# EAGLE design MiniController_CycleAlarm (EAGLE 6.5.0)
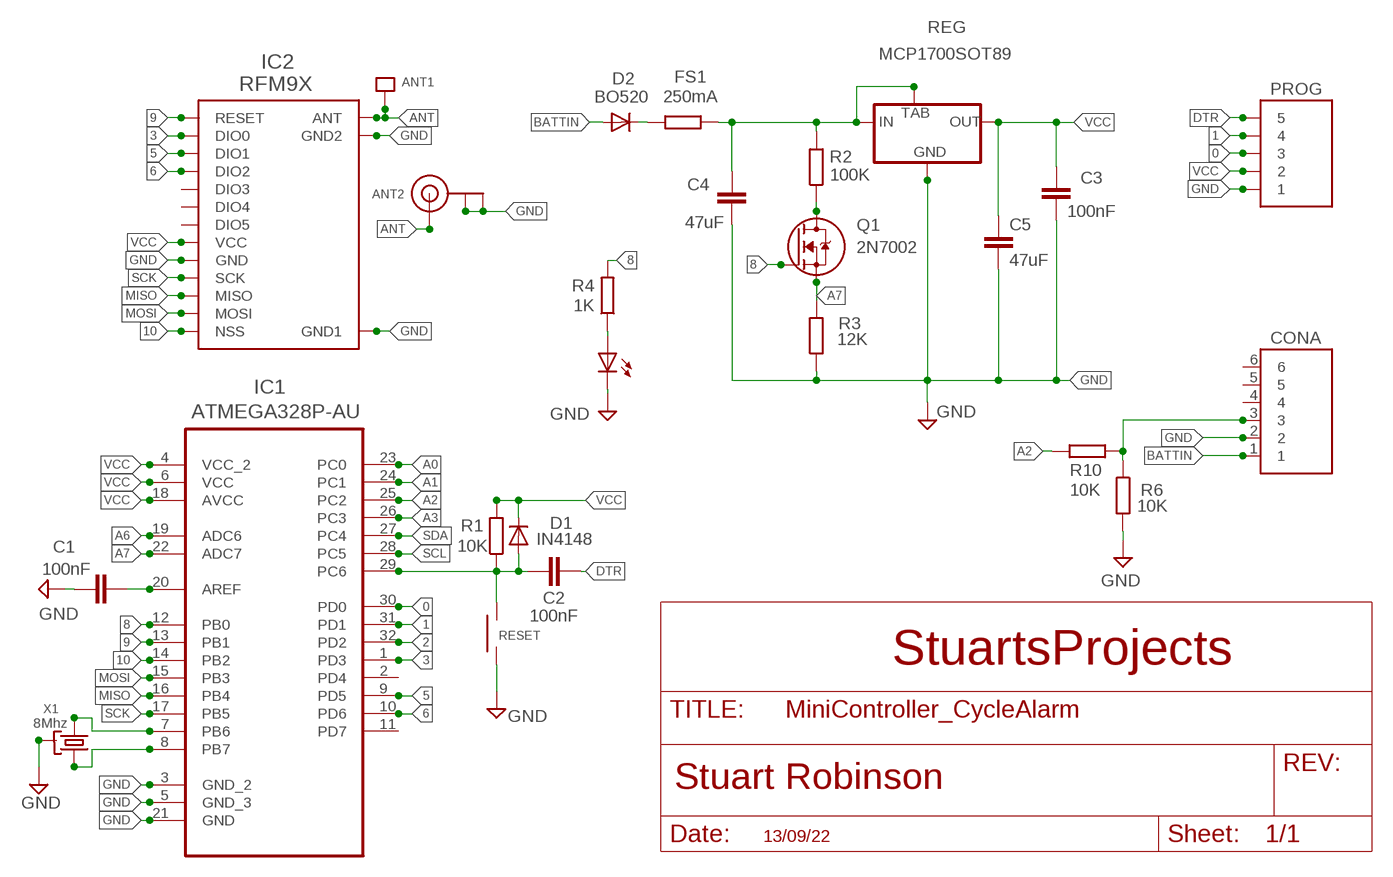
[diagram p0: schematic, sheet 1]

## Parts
ANT1  SINGLEPAD  [SINGLEPAD]
ANT2  ANTENNA_U.FL  [U.FL]
C1  100nF  C805_REDUCED  [C0805_REDUCED]
C2  100nF  C805_REDUCED  [C0805_REDUCED]
C3  100nF  C805_REDUCED  [C0805_REDUCED]
C4  47uF  C-EUC1206  [C1206]
C5  47uF  C-EUC1206  [C1206]
CONA  6X1BATPADS  [6X1_BATPADS]
D1  IN4148  DIODE-SOD123  [SOD123]
D2  BO520  DIODE-SOD123  [SOD123]
FS1  250mA  R-EU_R1206  [R1206]
IC1  ATMEGA328P-AU  [QFP80P900X900X120-32N]
IC2  RFM9X  RFM98  [RFM98]
L1  RED  LEDCHIPLED_0805  [CHIPLED_0805]
PROG  5X1  [5X1]
Q1  2N7002  [SOT23]
R1  10K  R0805_REDUCED  [R0805_REDUCED]
R2  100K  R0805_REDUCED  [R0805_REDUCED]
R3  12K  R0805_REDUCED  [R0805_REDUCED]
R4  1K  R0805_REDUCED  [R0805_REDUCED]
R6  10K  R0805_REDUCED  [R0805_REDUCED]
R10  10K  R0805_REDUCED  [R0805_REDUCED]
REG  MCP1700SOT89  [MCP1700SOT89]
RESET  SMTSWITCH_4_X_3  [SMTSWITCH_4_X_3]
X1  8Mhz  SMTRESONATOR3  [SMTRESONATOR3]

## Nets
0: IC1.30(PD0) PROG.3
1: IC1.31(PD1) PROG.4
2: IC1.32(PD2)
3: IC1.1(PD3) IC2.14(DIO0)
5: IC1.9(PD5) IC2.15(DIO1)
6: IC1.10(PD6) IC2.16(DIO2)
8: IC1.12(PB0) Q1.1(G) R4.2
9: IC1.13(PB1) IC2.6(RESET)
10: IC1.14(PB2) IC2.5(NSS)
A0: IC1.23(PC0)
A1: IC1.24(PC1)
A2: IC1.25(PC2) R10.2
A3: IC1.26(PC3)
A6: IC1.19(ADC6)
A7: IC1.22(ADC7) Q1.2(S) R3.2
ANT: ANT1.P$1 ANT2.3(SIGNAL) IC2.9(ANT)
BATTIN [POWER]: CONA.1 D2.A
DTR: C2.2 PROG.5
GND [POWER]: ANT2.1(GND) ANT2.2(GND) C1.2 C3.2 C4.2 C5.2 CONA.2 IC1.3(GND_2) IC1.5(GND_3) IC1.21(GND) IC2.1(GND) IC2.8(GND1) IC2.10(GND2) L1.C PROG.1 R3.1 R6.2 REG.1(GND) RESET.1 X1.G(GND)
MISO: IC1.16(PB4) IC2.2(MISO)
MOSI: IC1.15(PB3) IC2.3(MOSI)
N$2: IC1.8(PB7) X1.X1
N$3: C1.1 IC1.20(AREF)
N$5 [POWER]: D2.C FS1.2
N$6: L1.A R4.1
N$9: Q1.3(D) R2.1
N$11 [POWER]: C4.1 FS1.1 R2.2 REG.2(IN) REG.4(TAB)
N$13: CONA.3 R6.1 R10.1
N$16: IC1.7(PB6) X1.X2
RESET: C2.1 D1.A IC1.29(PC6) R1.1 RESET.2
SCK: IC1.17(PB5) IC2.4(SCK)
SCL: IC1.28(PC5)
SDA: IC1.27(PC4)
VCC [VDD]: C3.1 C5.1 D1.C IC1.4(VCC_2) IC1.6(VCC) IC1.18(AVCC) IC2.13(VCC) PROG.2 R1.2 REG.3(OUT)
Unconnected: CONA.4 CONA.5 CONA.6 IC1.2(PD4) IC1.11(PD7) IC2.7(DIO5) IC2.11(DIO3) IC2.12(DIO4)

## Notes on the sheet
- StuartsProjects
- 13/09/22

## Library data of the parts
ANT1 = LMA2:SINGLEPAD
ANT2 = adafruit:ANTENNA_U.FL: U.FL Antenna Connector
C1-C3 = resistor:C805_REDUCED
C4 C5 = resistor:C-EU: CAPACITOR, European symbol
CONA = My_Pin_Headers:6X1
D1 D2 = diode:DIODE-: DIODE
FS1 = resistor:R-EU_: RESISTOR, European symbol
IC1 = atmel:ATMEGA328P-AU: 8-bit Microcontroller with In-System Programmable Flash; MPN: ATMEGA328P-AU; OC_FARNELL: 1715486; OC_NEWARK: 14R4631; PACKAGE: TQFP-32; SUPPLIER: Atmel
IC2 = LMA2:RFM98
L1 = led:LED: LED
PROG = My_Pin_Headers:5X1
Q1 = LMA2:2N7002
R1-R4 R6 R10 = resistor:R0805_REDUCED
REG = LMA2:MCP1700SOT89
RESET = LMA2:SMTSWITCH_4_X_3
X1 = LMA2:SMTRESONATOR3

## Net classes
0 default: width 0.152 mm
1 POWER: width 0.508 mm
2 VDD: width 0.508 mm
3 gpspower: width 0.508 mm

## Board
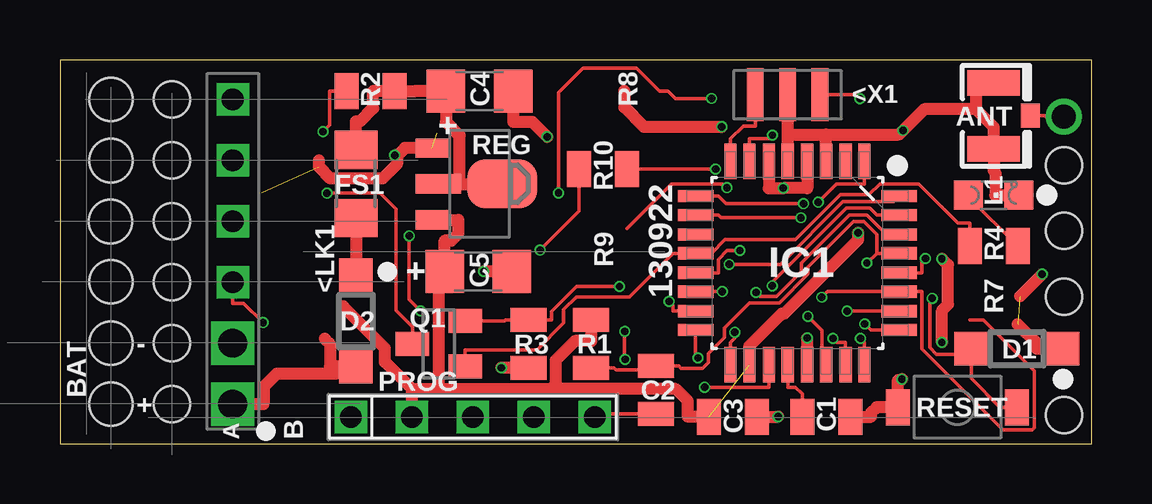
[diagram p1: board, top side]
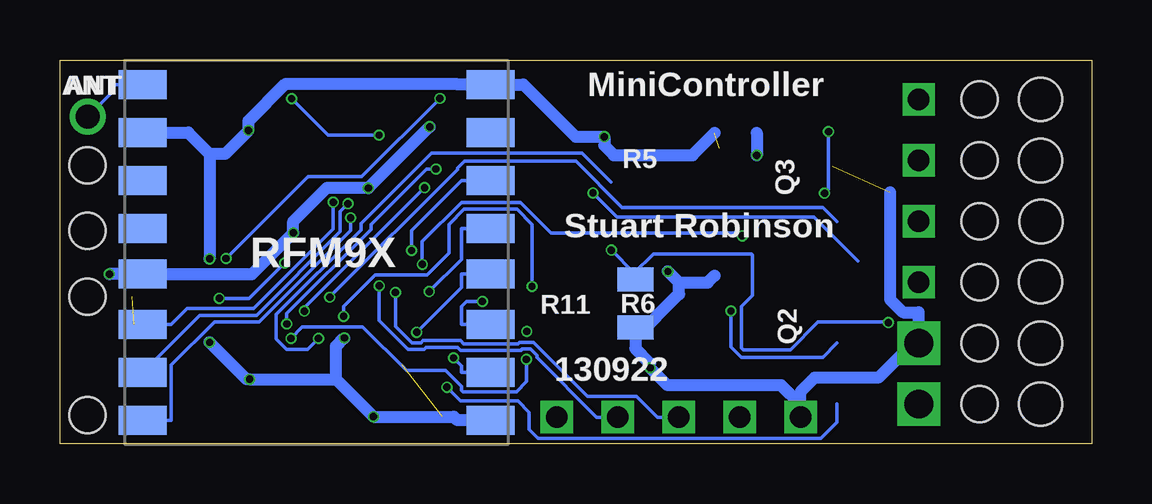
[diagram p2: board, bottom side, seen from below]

Size 43 x 16 mm. Coordinates in mm from the lower left corner, seen from the top.
Outline: 0,0 43,0 43,16 0,16 0,0
Copper layers (1*16): Top 0.035559375mm / dielectric 1.6mm / Bottom 0.035559375mm
Design rules "jlcpcb2layer *": minimum track width 5mil, minimum drill 12mil, track to track 5mil, track to pad 5mil, pad to pad 5mil, via to via 5mil, smd to smd 5mil, copper to edge 8mil, drill to drill 6mil, minimum pad ring 5mil, minimum via ring 3mil, stop-mask expansion 2.5mil, vias tented up to drill 1000mil, thermal gap 10mil
Holes 1.5 mm at 41.85,11.61 41.85,6.13 41.85,1.18 41.85,8.87 4.66,14.35 4.66,11.81 4.66,9.27 4.66,6.73 4.66,4.19 4.66,1.65
Holes 1.8 mm at 2.12,14.35 2.12,11.8 2.11,9.26 2.12,6.75 2.12,4.19 2.12,1.65
tRestrict: area 0,0 to 6.4,16
bRestrict: area 41.4,17.3 to 41.4,17.3; area 0,-0.1 to 6.4,16

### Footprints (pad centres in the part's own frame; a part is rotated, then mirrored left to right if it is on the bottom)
SINGLEPAD = drill 1: P$1 0,0
U.FL = smd 2.2 x 1.05: 1 0,1.375; 2 0,-1.375 | smd 0.8 x 1: 3 1.525,0
C0805_REDUCED = smd 1 x 1.5: 1 -1,0; 2 1,0
C1206 = smd 1.6 x 1.8: 1 -1.4,0; 2 1.4,0
6X1_BATPADS = drill 1.2 square: 1 -6.35,0; 2 -3.81,0 | drill 0.9 square: 3 -1.27,0; 4 1.27,0; 5 3.81,0; 6 6.35,0
SOD123 = smd 1.4 x 1.4: A 1.9,0; C -1.9,0
R1206 = smd 1.6 x 1.803: 1 -1.422,0; 2 1.422,0
QFP80P900X900X120-32N = smd 1.473 x 0.508: 1 -4.242,2.794; 2 -4.242,2.007; 3 -4.242,1.194; 4 -4.242,0.406; 5 -4.242,-0.406; 6 -4.242,-1.194; 7 -4.242,-2.007; 8 -4.242,-2.794; 17 4.242,-2.794; 18 4.242,-2.007; 19 4.242,-1.194; 20 4.242,-0.406; 21 4.242,0.406; 22 4.242,1.194; 23 4.242,2.007; 24 4.242,2.794 | smd 0.508 x 1.473: 9 -2.794,-4.242; 10 -2.007,-4.242; 11 -1.194,-4.242; 12 -0.406,-4.242; 13 0.406,-4.242; 14 1.194,-4.242; 15 2.007,-4.242; 16 2.794,-4.242; 25 2.794,4.242; 26 2.007,4.242; 27 1.194,4.242; 28 0.406,4.242; 29 -0.406,4.242; 30 -1.194,4.242; 31 -2.007,4.242; 32 -2.794,4.242
RFM98 = smd 2 x 1.2: 1 -7.25,7; 2 -7.25,5; 3 -7.25,3; 4 -7.25,0.9; 5 -7.25,-1; 6 -7.25,-3; 7 -7.25,-5; 8 -7.25,-7; 9 7.25,-7; 10 7.25,-5; 11 7.25,-3; 12 7.25,-1; 13 7.25,0.9; 14 7.25,3; 15 7.25,5; 16 7.25,7
CHIPLED_0805 = smd 1.2 x 1.2: A 0,-1.05; C 0,1.05
5X1 = drill 0.9 square: 1 -5.08,0; 2 -2.54,0; 3 0,0; 4 2.54,0; 5 5.08,0
SOT23 = smd 1 x 1.4: 1 -0.95,-1.1; 2 0.95,-1.1; 3 0,1.1
R0805_REDUCED = smd 1 x 1.5: 1 -1,0; 2 1,0
MCP1700SOT89 = smd 0.8 x 1.4: 1 -1.499,-1.981; 3 1.499,-1.981 | smd 0.8 x 1.9: 2 0,-1.727 | smd 2.032 x 2.921: 4 0,0.94
SMTSWITCH_4_X_3 = smd 1 x 1.5: 1 -2.48,0; 2 2.48,0
SMTRESONATOR3 = smd 0.7 x 2.2: G 0,0; X1 -1.35,0; X2 1.35,0

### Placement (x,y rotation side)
ANT1  41.85,13.63 0 top
ANT2  38.92,13.67 0 top
C1  31.94,1.12 0 top
C2  24.84,2.24 270 top
C3  28.05,1.12 0 top
C4  17.49,14.7 0 top
C5  17.44,7.18 0 top
CONA  7.2,8 90 top
D1  39.89,3.96 180 top
D2  12.34,5.11 270 top
FS1  12.34,10.83 270 top
IC1  30.74,7.53 270 top
IC2  32.31,7.97 180 bottom
L1  38.92,10.36 270 top
PROG  17.21,1.1 0 top
Q1  15.79,4.16 90 top
R1  22.14,4.16 90 top
R2  12.94,14.7 0 top
R3  19.53,4.16 90 top
R4  38.92,8.24 180 top
R6  19.02,5.85 270 bottom
R10  22.64,11.45 0 top
REG  17.5,10.83 270 top
RESET  37.41,1.52 0 top
X1  30.33,14.55 0 top

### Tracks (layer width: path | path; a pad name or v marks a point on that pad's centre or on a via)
0  (via drill 0.3 pad 0.46)
  Top 0.152: IC1.30 34.46,8.72 33.64,9.54 32.92,9.54 30.91,7.53 30.91,7.18 29.87,6.14 29.18,6.14 v29.02,6.3
  Bottom 0.152: 21.02,1.98 18.97,1.98 18.09,1.1 PROG.3 | 21.02,1.98 | 21.02,1.98 23.26,4.22 23.85,4.22 23.91,4.17 26.18,4.17 26.31,4.3 27.86,4.3 27.95,4.21 28.33,4.21 29.02,4.89 v29.02,6.3
1  (via drill 0.3 pad 0.46)
  Top 0.152: v29.69,6.58 29.69,6.73 32.78,9.82 33.76,9.82 34.04,9.54 IC1.31
  Bottom 0.152: v29.69,6.58 29.69,5.14 28.48,3.93 27.83,3.93 27.74,4.02 26.43,4.02 26.29,3.88 23.79,3.88 23.73,3.94 23.38,3.94 23.12,3.69 23.12,3.6 20.63,1.1 PROG.4
2  (via drill 0.3 pad 0.46)
  Top 0.152: v27.9,7.48 30.02,7.48 32.64,10.1 34.75,10.1 IC1.32 | v15.03,5.53 14.56,6 v14.56,8.66
  Bottom 0.152: v14.56,8.66 14.67,8.78 22.54,8.78 23.81,10.05 26.26,10.05 27.9,8.42 v27.9,7.48 | 10.62,4.19 11.21,3.6 14.6,3.6 15.03,4.04 v15.03,5.53
3  (via drill 0.3 pad 0.46)
  Top 0.152: v31.61,10.07 32.37,10.83 33.53,10.83 IC1.1
  Bottom 0.152: v31.61,10.07 31.61,8.94 34.92,5.63 37.7,5.63 38.36,4.97 IC2.14
5  (via drill 0.3 pad 0.46)
  Top 0.152: IC1.9 27.44,10.32 27.76,10 v31,10
  Bottom 0.152: IC2.15 37.18,5.35 34.81,5.35 31.31,8.84 31.31,9.68 v31,10
6  (via drill 0.3 pad 0.46)
  Top 0.152: v30.88,9.42 27.56,9.42 27.44,9.54 IC1.10
  Bottom 0.152: v30.88,9.42 30.88,8.88 34.69,5.07 36.56,5.07 38.36,3.27 38.36,0.97 IC2.16
8
  Top 0.152: Q1.1 16.89,3.91 19.89,3.91 21,5.02 21,5.59 21.53,6.12 23.74,6.12 25.56,7.94 IC1.12 27.16,7.94 27.72,8.5 30.65,8.5 32.53,10.38 33.73,10.38 34.18,10.83 35.8,10.83 37.44,9.19 37.92,9.19 R4.2
9  (via drill 0.3 pad 0.46)
  Top 0.152: v28.34,8.05 27.8,8.05 27.44,7.68 27.44,7.12 IC1.13
  Bottom 0.152: v28.34,8.05 28.34,8.89 26.26,10.97 IC2.6
10  (via drill 0.3 pad 0.46)
  Top 0.152: v27.61,6.34 27.44,6.34 IC1.14
  Bottom 0.152: v27.61,6.34 26.26,7.68 26.26,8.97 IC2.5
A0  (via drill 0.3 pad 0.46)
  Top 0.152: v32.22,4.38 32.38,4.23 32.75,4.23 IC1.23
  Bottom 0.152: v32.22,4.38 32.68,3.93 33.55,3.93 33.98,4.37 33.98,5.38 30.45,8.91 30.45,9.17 27.51,12.11 21.24,12.11 20.04,10.91
A1  (via drill 0.3 pad 0.46)
  Top 0.152: v23.54,4.68 23.54,3.52 v23.56,3.51 | v33.37,4.39 33.53,4.23 IC1.24
  Bottom 0.152: 23.42,4.8 v23.54,4.68 | v23.56,3.51 23.56,2.59 23.98,2.17 26.2,2.17 26.26,2.23 26.26,2.38 26.93,3.04 28.56,3.04 30.38,4.86 32.9,4.86 v33.37,4.39
A2  (via drill 0.3 pad 0.46)
  Top 0.152: R10.2 v27.33,11.45 | v33.55,4.99 33.8,4.74 IC1.25
  Bottom 0.152: v33.55,4.99 33.55,5.42 30.03,8.94 30.03,9.13 27.72,11.45 v27.33,11.45
A3  (via drill 0.3 pad 0.46)
  Top 0.152: 23.64,8.97 25.5,10.83 27.64,10.83 v27.8,10.67 | v32.81,5.52 IC1.26
  Bottom 0.152: v32.81,5.52 32.81,5.66 v27.8,10.67
A6  (via drill 0.3 pad 0.46)
  Top 0.152: v26.87,2.35 29.55,2.35 IC1.19
  Bottom 0.152: 10.62,1.65 10.62,0.88 11.28,0.22 23.08,0.22 23.45,0.6 23.45,1.31 23.91,1.77 26.29,1.77 v26.87,2.35
A7  (via drill 0.3 pad 0.46)
  Top 0.152: v31.18,5.31 31.77,4.72 31.77,3.45 IC1.22 | v23.32,6.56 21.53,6.56 20.48,5.51 20.48,5.16 R3.2 19.05,5.16 18.58,5.16 18.53,5.11 Q1.2
  Bottom 0.152: v23.32,6.56 23.32,9.14 23.96,9.77 26.15,9.77 26.78,9.14 26.78,7.95 27.71,7.03 29.87,7.03 31.18,5.72 v31.18,5.31
ANT
  Top 0.152: ANT1.P$1 41.09,13.63 41.05,13.67 ANT2.3
  Bottom 0.152: IC2.9 40.76,14.97 40.76,14.72 ANT1.P$1
BATTIN
  Top 0.508: CONA.1 8.48,1.65 8.48,2.36 9.03,2.91 11.5,2.91 11.8,3.21 | 11.8,3.21 11.26,3.21 11.26,4.15 11.04,4.37 | D2.A 11.8,3.21
DTR
  Top 0.152: PROG.5 22.43,1.24 23.89,1.24 C2.2
GND  (via drill 0.3 pad 0.46)  (2 unrouted)
  Top 0.508: IC1.21 v31.15,4.41 | C3.2 v29.93,1.12 | C5.2 v17.66,7.18 | v20.31,12.79 19.68,13.42 18.89,13.42 C4.2 | 14.04,12 14.04,11.65 13.46,11.06 11.28,11.06 10.8,11.54 10.8,11.81 | 14.04,12 14.38,12.33 14.44,12.33 REG.1 | 14.04,12 14.01,12.03 v13.95,12.03 | v36.76,4.22 36.76,5.55 37.02,5.81 37.02,7.45 v36.76,7.71 | 30.33,12.89 30.33,13.06 30.33,13.07 X1.G | IC1.5 30.33,12.89 | 30.33,12.89 31.93,12.89 | 31.93,12.89 34.97,12.89 v35.14,13.06 36.02,13.94 38.18,13.94 | C1.2 33.82,1.12 33.82,1.29 34.05,1.52 RESET.1 34.93,2.65 35.06,2.65 v35.09,2.68 | IC1.3 31.93,12.89 | L1.C 38.99,10.36 38.99,11.32 38.92,11.39 ANT2.2 38.92,13.2 38.18,13.94 | ANT2.1 38.18,15.04 38.18,13.94 | R3.1 v18.4,3.16
  Bottom 0.508: 15.71,12.95 16.63,12.03 19.91,12.03 20.31,12.43 v20.31,12.79 21.5,12.79 23.68,14.97 IC2.8 26.44,14.97 26.48,15.01 33.59,15.01 35.14,13.45 v35.14,13.06 36.12,12.08 36.76,12.08 | 31.5,2.68 31.5,4.06 v31.15,4.41 | 31.5,2.68 v29.93,1.12 26.59,1.12 26.44,0.97 IC2.1 | 31.5,2.68 v35.09,2.68 35.23,2.68 v36.76,4.22 | 17.19,6.71 v17.66,7.18 | 19.02,4.41 17.19,6.24 17.19,6.71 | 17.19,6.71 16.01,6.71 15.71,7.01 | 19.02,4.41 19.02,3.97 18.4,3.35 v18.4,3.16 17.68,2.44 12.94,2.44 12.13,1.63 | R6.2 19.02,4.41 | 12.13,1.63 12.13,2.16 11.54,2.74 8.89,2.74 7.2,4.43 | PROG.1 12.13,1.63 | 13.95,12.95 v13.95,12.03 | CONA.2 7.2,4.43 | 7.2,4.43 7.2,4.47 7.2,5.47 7.86,5.47 8.4,6.02 8.4,10.47 | IC2.10 37.65,12.97 36.76,12.08 | 36.76,12.08 v36.76,7.71
MISO  (via drill 0.3 pad 0.46)
  Top 0.152: IC1.16 26.5,3.67 v26.59,3.57
  Bottom 0.152: v26.59,3.57 26.26,3.24 26.26,2.97 IC2.2
MOSI  (via drill 0.3 pad 0.46)
  Top 0.152: IC1.15 25.56,5.52 25.56,5.76 v25.39,5.93
  Bottom 0.152: IC2.3 26.26,4.97 26.26,5.71 26.05,5.93 v25.39,5.93
N$2
  Top 0.152: X1.X1 28.98,13.25 28.48,13.25 27.95,12.71 IC1.8
N$3
  Top 0.152: IC1.20 30.33,2.35 30.66,2.35 30.94,2.07 C1.1
N$5
  Top 0.508: FS1.2 D2.C
N$6
  Top 0.152: R4.1 37.87,10.29 L1.A
N$9  (via drill 0.3 pad 0.46)
  Top 0.152: R2.1 11.24,14.7 11.24,13.29 v10.96,13.01 | v11.13,10.44 13.35,10.44 14.01,9.78 14.01,5.55 14.69,4.86 Q1.3
  Bottom 0.152: v10.96,13.01 10.96,10.6 v11.13,10.44
N$11
  Top 0.508: FS1.1 12.34,13.43 12.51,13.43 13.06,13.99 13.06,14.7 R2.2 14.82,14.7 C4.1 16.09,13.42 16.66,12.85 16.66,10.83 | REG.2 16.66,10.83 | 16.66,10.83 REG.4
N$13  (via drill 0.3 pad 0.46)
  Top 0.152: R10.1 21.64,9.69 v20.02,8.07 | v8.47,5.04 7.66,5.85 7.2,5.85 CONA.3
  Bottom 0.152: 19.07,7.12 18.27,7.92 14.17,7.92 14.13,7.87 14.13,6.19 14.58,5.73 14.58,3.99 14.5,3.91 12.56,3.91 11.4,5.07 8.49,5.07 v8.47,5.04 | 19.07,7.12 19.33,6.85 R6.1 | v20.02,8.07 19.07,7.12
N$16  (via drill 0.3 pad 0.46)
  Top 0.152: X1.X2 33.18,14.55 v33.34,14.39 | v29.69,12.86 29.54,12.71 28.73,12.71 IC1.7
  Bottom 0.152: v29.69,12.86 31.82,12.86 v33.34,14.39
RESET  (via drill 0.3 pad 0.46)
  Top 0.152: 34.04,7.94 34.04,8.72 33.51,9.26 33.08,9.26 31.19,7.36 31.19,7.07 29.99,5.87 28.74,5.87 27.69,4.82 27.69,4.43 27.02,3.76 27.02,3.4 26.77,3.14 25.89,3.14 25.79,3.24 C2.1 24.68,3.08 23.18,3.08 23.09,3.16 R1.1 | 37.99,3.73 36.54,3.73 36.25,4.01 36.25,5.96 v36.36,6.06 | 37.99,3.73 37.99,2.72 39.19,1.52 RESET.2 | D1.A 37.99,3.73 | v33.64,7.53 34.04,7.94 | IC1.29 34.04,7.94
  Bottom 0.152: v36.36,6.06 35.11,6.06 v33.64,7.53
SCK  (via drill 0.3 pad 0.46)
  Top 0.152: IC1.17 27.95,4.23 28.13,4.41 v28.13,4.64
  Bottom 0.152: IC2.4 26.26,7.07 26.26,6.5 v28.13,4.64
SCL  (via drill 0.3 pad 0.46)
  Top 0.152: v20.79,10.46 20.79,14.63 21.81,15.65 24.04,15.65 24.99,14.7 25.34,14.7 25.65,14.4 v27.16,14.4 | IC1.28 35.92,7.12 35.92,7.56 v36.08,7.72
  Bottom 0.152: 9.74,7.61 11.58,9.45 19.78,9.45 v20.79,10.46 | v36.08,7.72 32.67,11.13 30.43,11.13 v27.16,14.4
SDA  (via drill 0.3 pad 0.46)
  Top 0.152: v31.76,6.1 31.99,6.34 IC1.27 35.45,6.34 35.92,6.34 35.92,3.95 39.3,0.57 40.53,0.57 40.61,0.65 40.61,3.04 38.49,5.16 37.92,5.16
  Bottom 0.152: 10.62,9.27 11.2,9.85 19.56,9.85 21.49,11.78 26.14,11.78 26.42,11.5 26.42,11.44 v31.76,6.1
VCC  (via drill 0.3 pad 0.46)  (2 unrouted)
  Top 0.508: IC1.18 28.73,4.07 30.08,5.41 30.18,5.41 33.27,8.5 v33.27,8.79 | 14.67,2.28 13.55,3.4 13.55,3.98 11.8,5.72 | C3.1 26.17,1.12 26.17,1.78 25.67,2.28 20.85,2.28 20.66,2.47 | 23.52,14.7 23.52,14.03 24.33,13.21 v27.59,13.21 | R1.2 22.14,4.28 21.46,4.28 20.66,3.48 20.66,2.47 | REG.3 16.6,9.33 16.6,8.74 16.32,8.46 16.04,8.46 C5.1 15.79,6.93 15.79,2.28 | IC1.4 31.15,10.65 v30.15,10.65 29.55,10.65 IC1.6 | 40.01,6.14 v40.94,7.07 | 39.92,4.98 40.71,4.19 40.71,3.96 D1.C | PROG.2 14.67,2.28 | 14.67,2.28 15.79,2.28 | 15.79,2.28 20.47,2.28 20.66,2.47
  Bottom 0.508: v27.59,13.21 v30.15,10.65 30.17,10.68 31.86,10.68 33.27,9.26 v33.27,8.79 34.99,7.07 IC2.13 v40.94,7.07

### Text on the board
tPlace: - | BAT | +
bPlace: ANT | 130922
tNames: C4 | R8 | R2 | + | <X1 | ANT | R10 | REG | FS1 | 130922 | L1 | <LK1 | R9 | + | R4 | C5 | IC1 | Q1 | D2 | R3 | R7 | R1 | D1 | C2 | PROG | C1 | RESET | A | B | C3
bNames: MiniController | ANT | Q3 | R5 | Stuart Robinson | RFM9X | Q2 | R6 | R11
